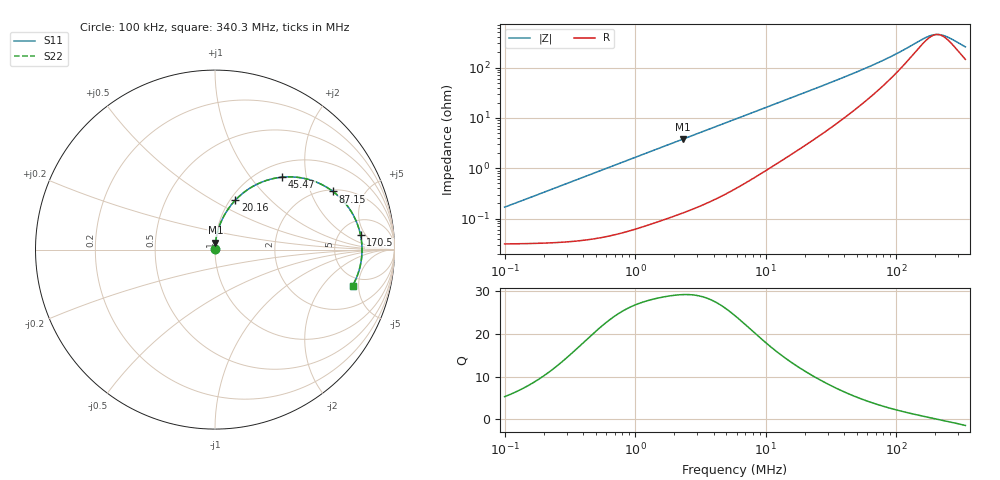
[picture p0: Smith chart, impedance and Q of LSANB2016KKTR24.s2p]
! LSANB2016KKTR24  S-PARAMETER MODEL  ( General Type )
! Model Generated by TAIYO YUDEN Corporation (http://www.ty-top.com)
! Version 3.0
! TAIYO YUDEN Control No. 160323NG38SB-FKC
! Copyright(c) 2013 TAIYO YUDEN CO.,LTD. All Rights Reserved.
! Product Description (link to TY-COMPAS)
! https://ds.yuden.co.jp/TYCOMPAS/or/detail?pn=LSANB2016KKTR24M&u=M
! Products Name : Inductors
! Characteristics :
!  Inductance : 0.24 uH , SRF(min) : -Hz , DC Resistance(max) : 0.037 Ohm
!  Rated Current : Saturation :4200 mA , Temp Rise : 3000 mA (40 degC)
!  Case Size : 2.0 x 1.6 / 0.079 x 0.063 [mm/inch] , Thickness : 1 / 0.039 [mm/inch]
!  (Conditions: Temperature = 25 degC , DC Bias Current/Voltage = 0A / 0V)
! External Node Assignments :
!  1  o---GGG---o  2
! GND o---------o GND
! Frequency Range : 0.1MHz  -  340.31115MHz  [ 402 STEP ]
# MHz S RI R 50
! Freq[MHz].  S11 Real  S11 Imag  S21 Real  S21 Imag  S12 Real  S12 Imag  S22 Real  S22 Imag
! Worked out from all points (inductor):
!   401 points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, 100 kHz to 340.3 MHz, reference 50 ohm
!   read as one part in series: L = 264 nH near 104.2 kHz
!   highest Q = 29.2 at 2.337 MHz (marker M1), where L = 258 nH
!   self-resonance near 206.9 MHz
!   S11 on the Smith chart (normalised r, x): 100 kHz: 1.00, +0.00; 20.16 MHz: 1.06, +0.64; 45.47 MHz: 1.26, +1.45; 87.15 MHz: 2.08, +2.91; 170.5 MHz: 7.98, +3.80; 340.3 MHz: 3.90, -4.24
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0.1  0.000317 0.00166  0.9997 -0.00166  0.9997 -0.00166  0.000317 0.00166
0.390471  0.000409 0.00645  0.9996 -0.00645  0.9996 -0.00645  0.000409 0.00645
1.524679  0.00149 0.0248  0.9985 -0.0248  0.9985 -0.0248  0.00149 0.0248
2.336695  0.00273 0.0378  0.9973 -0.0378  0.9973 -0.0378  0.00273 0.0378
5.953437  0.0129 0.094  0.9871 -0.094  0.9871 -0.094  0.0129 0.094
12.1285  0.0467 0.1819  0.9533 -0.1819  0.9533 -0.1819  0.0467 0.1819
15.79767  0.0745 0.2277  0.9255 -0.2277  0.9255 -0.2277  0.0745 0.2277
20.16272  0.1131 0.2752  0.8869 -0.2752  0.8869 -0.2752  0.1131 0.2752
22.77862  0.1384 0.2999  0.8616 -0.2999  0.8616 -0.2999  0.1384 0.2999
32.18341  0.2363 0.3653  0.7637 -0.3653  0.7637 -0.3653  0.2363 0.3653
45.47124  0.3731 0.4035  0.6269 -0.4035  0.6269 -0.4035  0.3731 0.4035
53.50253  0.4465 0.404  0.5535 -0.404  0.5535 -0.404  0.4465 0.404
62.95234  0.5209 0.3908  0.4791 -0.3908  0.4791 -0.3908  0.5209 0.3908
74.0712  0.5923 0.3637  0.4077 -0.3637  0.4077 -0.3637  0.5923 0.3637
87.15392  0.6569 0.324  0.3431 -0.324  0.3431 -0.324  0.6569 0.324
88.94399  0.6644 0.3183  0.3356 -0.3183  0.3356 -0.3183  0.6644 0.3183
123.1379  0.7609 0.209  0.2391 -0.209  0.2391 -0.209  0.7609 0.209
170.4774  0.8111 0.08  0.1889 -0.08  0.1889 -0.08  0.8111 0.08
196.5507  0.8187 0.0212  0.1813 -0.0212  0.1813 -0.0212  0.8187 0.0212
222.051  0.8183 -0.0295  0.1817 0.0295  0.1817 0.0295  0.8183 -0.0295
250.8597  0.8116 -0.08  0.1884 0.08  0.1884 0.08  0.8116 -0.08
340.3111  0.7665 -0.2018  0.2335 0.2018  0.2335 0.2018  0.7665 -0.2018
